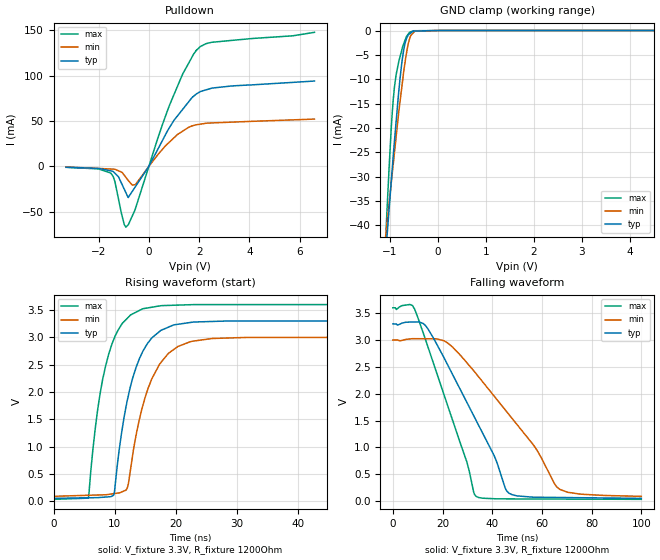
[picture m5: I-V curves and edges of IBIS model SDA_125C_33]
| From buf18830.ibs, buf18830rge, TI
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|   SDA_33 Model
[Model] SDA_125C_33
|Signals SDA(15)
Model_type   I/O_open_drain
Polarity   Non-Inverting
Enable   Active-Low
Vinl = 0.99
Vinh = 2.31
Vmeas = 1.65
Vref = 1.65
Cref = 0pF
Rref = 10000
| Rpullup to DVDD = 1k
|   typ   min   max
|   (nom PVT)   (slow PVT)   (Fast PVT)
|   Output LOW
|C_comp   9.86462E-13   8.35757E-13   1.26497E-12
|   Output HIGH
C_comp   1.12741E-12   9.81932E-13   1.3179E-12
| Where   nom PVT is  Nominal Process, 3.3V, 67C
|   Fast PVT is Strong Process, 3.6V, -40C
|   Slow PVT is Weak Process, 3.0V, 125C
[Model Spec]   |3.3V model
Vinl   0.99   0.9   1.08
Vinh   2.31   2.1   2.52
|Vinl = 0.3 X DVDD
|Vinh = 0.7 X DVDD
[Voltage Range]   3.3   3   3.6
|Operating Temperature   27   85   -40
[Temperature Range]   67   125   -40
[Pullup Reference]   3.3   3   3.6
[Pulldown Reference]   0   0   0
[Power Clamp Reference]   3.3   3   3.6
[GND Clamp Reference]   0   0   0
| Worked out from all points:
|   slope of the pulldown table from 0 to 0.495 V, typ, clamps not added: 19 ohm
|   GND clamp passes 1 mA (typ) near -0.62 V on its own axis
|   falling waveform, V_fixture 3.3V, R_fixture 1200Ohm: 20-80 % time 21.2ns typ, 28.5ns min, 15.6ns max; typ from 3.3 V to 0.051 V
|   rising waveform, V_fixture 3.3V, R_fixture 1200Ohm: 20-80 % time 3.74ns typ, 4.21ns min, 3.33ns max; typ from 0.051 V to 3.3 V
[Pulldown]
|   Voltage   I(typ)   I(min)   I(max)
-3.3V     -960.2uA   -657.3uA   -1.057mA
-1.508V   -5.011mA   -2.934mA   -7.667mA
-1.355V   -7.475mA   -3.128mA   -16.42mA
-1.095V   -18.25mA   -6.305mA   -51.39mA
-913.6mV  -29.04mA   -12.14mA   -66.93mA
-824mV    -34.36mA   -15.35mA   -64.39mA
-547.8mV  -22.83mA   -20.24mA   -47.6mA
828.8mV   43.06mA    27mA       67.83mA
1.352V    63mA       38.89mA    101.9mA
1.888V    79.64mA    45.75mA    127.6mA
2.507V    86.11mA    47.8mA     136.6mA
6.59V     93.92mA    52.04mA    147.6mA
[GND Clamp]
|   Voltage   I(typ)   I(min)   I(max)
-3.3V     -358.4mA   -267.9mA   -579.2mA
-1.109V   -48.59mA   -43.88mA   -47.16mA
-1.072V   -43.54mA   -40.43mA   -38.92mA
-1.06V    -41.98mA   -39.35mA   -36.53mA
-974.2mV  -31.03mA   -31.33mA   -20.14mA
-907.5mV  -22.78mA   -25.12mA   -11.61mA
-747.5mV  -6.177mA   -11.13mA   -3.761mA
-685.4mV  -2.606mA   -6.493mA   -1.976mA
-594.7mV  -716.2uA   -1.806mA   -394.2uA
-480.9mV  -111.7uA   -126.3uA   -44.67uA
-4.065mV  -1.395uA   0A         -37.37nA
6.59V     0A         0A         0A
[POWER Clamp]
|   SCR cell for ESD function. Effects occurr above VDD x 2
|   Voltage   I(typ)   I(min)   I(max)
-3.3V     0A         0A         0A
0V        0A         0A         0A
6.6V      0A         0A         0A
[Ramp]
R_load = 1200
|   typ   min   max
dV/dt_r   1.94916/3.73652e-009   1.7467/4.16272e-009   2.13988/3.33144e-009
dV/dt_f   1.94916/2.12037e-008   1.7467/2.85383e-008   2.13988/1.56234e-008
[Falling Waveform]
V_fixture = 3.3V
V_fixture_min = 3V
V_fixture_max = 3.6V
R_fixture = 1200Ohm
C_fixture = 0F
|   Time   V(typ)   V(min)   V(max)
0s        3.3V       3V         3.6V
8.776ns   3.336V     3.024V     3.574V
13.1ns    3.271V     3.023V     3.014V
20.66ns   2.664V     2.984V     1.974V
29.8ns    1.838V     2.576V     726.5mV
33.47ns   1.508V     2.376V     91.16mV
46.92ns   143.2mV    1.602V     41.57mV
56.75ns   73.27mV    1.036V     40.08mV
67.13ns   68.01mV    221.5mV    38.51mV
100ns     51.39mV    88.83mV    33.53mV
[Rising Waveform]
V_fixture = 3.3V
V_fixture_min = 3V
V_fixture_max = 3.6V
R_fixture = 1200Ohm
C_fixture = 0F
|   Time   V(typ)   V(min)   V(max)
0s        51.39mV    88.83mV    33.53mV
5.697ns   61.71mV    107.7mV    56.04mV
7.646ns   67.68mV    114.1mV    1.984V
9.82ns    108.3mV    136.8mV    2.949V
12.1ns    1.859V     250.6mV    3.35V
14.51ns   2.718V     1.707V     3.517V
16.09ns   2.987V     2.239V     3.55V
18.74ns   3.182V     2.699V     3.583V
26ns      3.289V     2.978V     3.598V
100ns     3.3V       3V         3.6V
